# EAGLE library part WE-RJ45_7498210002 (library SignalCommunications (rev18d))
WE-RJ45 LAN Transformer Order Code 7498210002 Design SMD xBase-T 10/100 Base-T Ports 1x1 Application Standard Tab Position DOWN LED (Left-Right) NO EMI Fingers No Details see: http://katalog.we-online.de/en/pbs/WE-LAN-RJ45 Created by Yingchun Shan 2016 (C) Wurth Elektronik
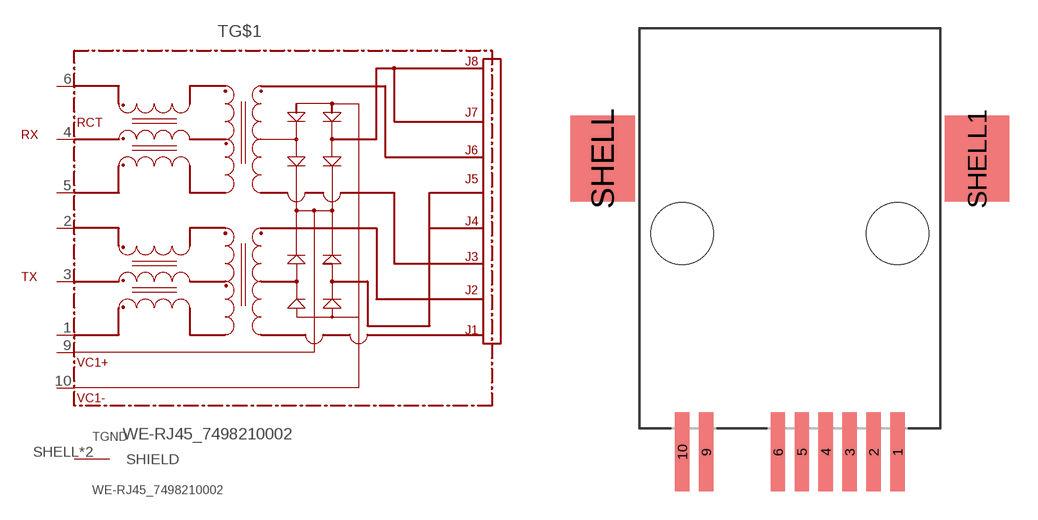
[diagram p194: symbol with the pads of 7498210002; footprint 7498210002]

Designator prefix T; gates G$1=7498210002 GND=SHIELD

## WE-RJ45_7498210002  [7498210002]
1  G$1:1
2  G$1:2
3  G$1:3
4  G$1:4
5  G$1:5
6  G$1:6
9  G$1:VC1+  pwr
10  G$1:VC1-  pwr
SHELL  GND:SHIELD  pas
SHELL1  GND:SHIELD  pas

## Footprint 7498210002 (pad centres in mm)
smd 0.76 x 4.18: 1 5.715,-11.61; 2 4.445,-11.61; 3 3.175,-11.61; 4 1.905,-11.61; 5 0.635,-11.61; 6 -0.635,-11.61; 9 -4.445,-11.61; 10 -5.715,-11.61
smd 3.42 x 4.58: SHELL -9.94,3.97; SHELL1 9.94,3.97
hole 3.3 at 5.715,0
hole 3.3 at -5.715,0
